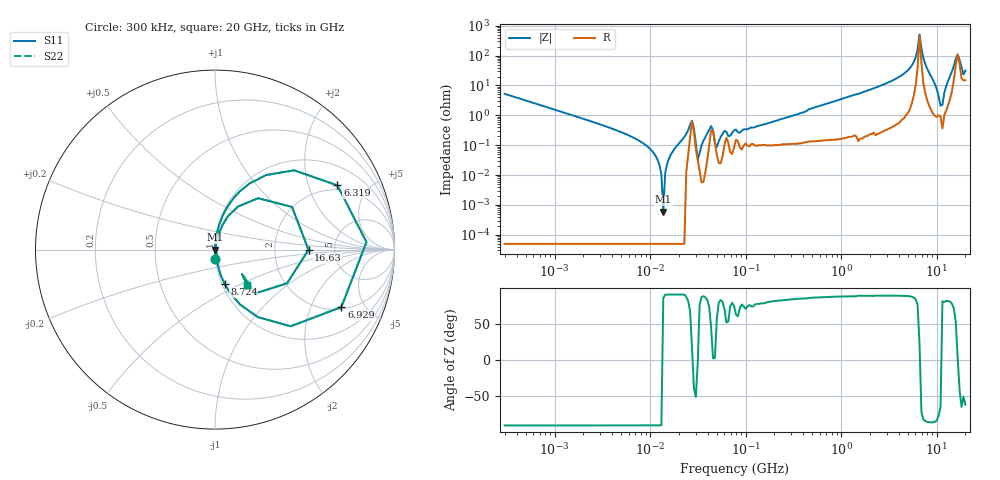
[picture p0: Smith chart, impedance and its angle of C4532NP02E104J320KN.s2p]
! S-parameter Generated by TDK Corporation
! Copyright(C) 2015 TDK Corporation.
! All Rights Reserved.
! TDK P/N: C4532NP02E104J320KN (Multilayer Ceramic Chip Capacitors)
! Property: C=100nF
! Size(LxWxT): 4.5x3.2x3.2mm, 0.177x0.126x0.126inches
! Model Type: s2p (Touchstone File Format Version 1.0)
! Frequency: DC=Yes Start=0.3MHz Stop=20000MHz 243points Log-sweep
! Note:
! Model Generated on Jun. 23, 2015
! Hash(MD5):
! Port Assignments:
!  1 ---| |--- 2
! Applicable Conditions:
!  Temperature = 25 degC
!  DC Bias Voltage = 0 V
!  Small Signal Operation
! Terms and conditions regarding TDK Simulation Models
! (1)This simulation model is being provided solely for informational purposes. Please refer to the specifications of the products in terms of detailed characteristics of such products.
! (2)In no event shall TDK Corporation of any of its subsidiaries be liable for any loss or damage arising, directly or indirectly,
!  From any information contained in this simulation model, including, but not limited to loss or damages arising from any inaccuracies, omissions or errors in connection with such information.
! (3)Any and all copyrights on this simulation model are owned by TDK Corporation.
!  Duplication or redistribution of this simulation model without prior written permission from TDK Corporation is prohibited.
! (4)This simulation model is subject to any modification or change without any prior notice.
! (5)Neither TDK Corporation nor any of its subsidiaries shall make any warranty, express or implied,
!  Including but not limited to the correctness, implied warranties of merchantability and fitness for a particular purpose with respect to this simulation models.
! (6)The use of this simulation model shall be deemed to have consented to the terms and conditions hereof.
# MHz S MA R 50
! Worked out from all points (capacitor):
!   242 points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, 300 kHz to 20 GHz, reference 50 ohm
!   read as one part in series: C = 101 nF near 314.2 kHz
!   lowest |Z| = 601 uohm at 13.76 MHz (marker M1)
!   series resonance near 13.72 MHz, so ESL is about 1.3 nH
!   S11 on the Smith chart (normalised r, x): 300 kHz: 1.00, -0.10; 6.319 GHz: 1.77, +3.12; 6.929 GHz: 2.11, -3.37; 8.724 GHz: 1.03, -0.41; 16.63 GHz: 3.18, -0.01; 20 GHz: 1.30, -0.56
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0.3  0.05234 -87.0  0.9986 3.0  0.9986 3.0  0.05234 -87.0
1.985118  0.007729 -89.8  0.9999 0.4  0.9999 0.4  0.007729 -89.8
7.555385  0.001464 -92.4  0.9999 0.1  0.9999 0.1  0.001464 -92.4
12.54397  0.0002297 -108.8  0.9999 0.0  0.9999 0.0  0.0002297 -108.8
13.75522  7.495e-05 175.2  0.9999 -0.0  0.9999 -0.0  7.495e-05 175.2
27.46064  0.006629 18.3  0.9937 -0.1  0.9937 -0.1  0.006629 18.3
31.53257  0.0003287 0.6  0.9997 0.0  0.9997 0.0  0.0003287 0.6
43.53844  0.004367 45.2  0.9969 -0.2  0.9969 -0.2  0.004367 45.2
49.99442  0.0008753 57.6  0.9995 -0.0  0.9995 -0.0  0.0008753 57.6
60.11549  0.003011 69.7  0.999 -0.2  0.999 -0.2  0.003011 69.7
79.26541  0.00332 62.3  0.9985 -0.2  0.9985 -0.2  0.00332 62.3
500.8786  0.0175 84.6  0.9985 -1.0  0.9985 -1.0  0.0175 84.6
3165.055  0.1275 81.1  0.9883 -7.3  0.9883 -7.3  0.1275 81.1
5254.842  0.3526 66.9  0.9208 -20.6  0.9208 -20.6  0.3526 66.9
6318.653  0.7699 27.7  0.476 -48.1  0.476 -48.1  0.7699 27.7
6616.689  0.8449 2.9  0.1656 -19.5  0.1656 -19.5  0.8449 2.9
6928.783  0.7734 -24.5  0.4316 46.7  0.4316 46.7  0.7734 -24.5
8724.45  0.1986 -74.3  0.9655 11.4  0.9655 11.4  0.1986 -74.3
11503.64  0.02243 79.5  0.9961 -1.3  0.9961 -1.3  0.02243 79.5
12614.44  0.09559 76.0  0.9812 -5.4  0.9812 -5.4  0.09559 76.0
16632.79  0.5211 -0.1  0.4789 -0.5  0.4789 -0.5  0.5211 -0.1
20000  0.2668 -48.0  0.8452 13.6  0.8452 13.6  0.2668 -48.0
